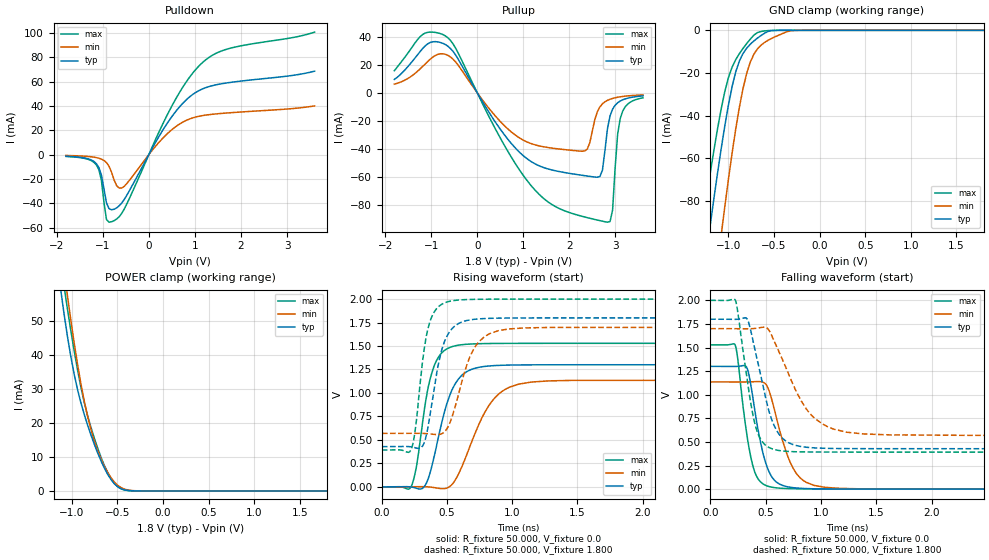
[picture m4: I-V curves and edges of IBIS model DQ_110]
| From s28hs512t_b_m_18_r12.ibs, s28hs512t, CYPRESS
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|   Model DQ_110
[Model] DQ_110
Model_type I/O
Polarity   Non-Inverting
Enable   Active-High
Vinl =  0.630V
Vinh =  1.170V
|Ac timing Thresholds
Vmeas =  0.900V
Cref =  15.000pF
C_comp   5.334pF   5.23pF   5.767pF
[Temperature Range]   25.000   0.125k   -40.000
[Voltage Range]   1.800V   1.700V   2.000V
[Pullup Reference]   1.800V   1.700V   2.000V
[Pulldown Reference]   0.0V   0.0V   0.0V
[POWER Clamp Reference]   1.800V   1.700V   2.000V
[GND Clamp Reference]   0.0V   0.0V   0.0V
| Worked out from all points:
|   slope of the pulldown table from 0 to 0.27 V, typ, clamps not added: 14.9 ohm
|   slope of the pullup table from 0 to 0.27 V, typ, clamps not added: 18.3 ohm
|   GND clamp passes 1 mA (typ) near -0.59 V on its own axis
|   POWER clamp passes 1 mA (typ) near -0.48 V on its own axis
|   rising waveform, R_fixture 50.000, V_fixture 0.0: 20-80 % time 151ps typ, 225ps min, 111ps max; typ from 0 V to 1.3 V
|   rising waveform, R_fixture 50.000, V_fixture 1.800: 20-80 % time 113ps typ, 158ps min, 87.3ps max; typ from 0.428 V to 1.8 V
|   falling waveform, R_fixture 50.000, V_fixture 0.0: 20-80 % time 131ps typ, 181ps min, 109ps max; typ from 1.3 V to 0 V
|   falling waveform, R_fixture 50.000, V_fixture 1.800: 20-80 % time 172ps typ, 292ps min, 127ps max; typ from 1.8 V to 0.428 V
[Pulldown]
|Voltage   I(typ)   I(min)   I(max)
-1.8V     -1.334mA   -724.2uA   -1.502mA
-1.14V    -7.446mA   -2.454mA   -8.441mA
-1.03V    -16.88mA   -3.691mA   -21.21mA
-920mV    -39.73mA   -6.551mA   -53.37mA
-755mV    -44.96mA   -20.8mA    -54.34mA
-645mV    -42.15mA   -27.51mA   -51.1mA
-535mV    -36.94mA   -26.09mA   -44.85mA
510mV     31.81mA    20.83mA    40.71mA
840mV     46.04mA    28.63mA    61.36mA
1.17V     54.13mA    32.13mA    75.91mA
1.775V    59.42mA    34.47mA    87.58mA
3.6V      68.65mA    40.07mA    100.8mA
[Pullup]
|Voltage   I(typ)   I(min)   I(max)
-1.8V     9.461mA    6.095mA    15.71mA
-1.185V   31.57mA    18.73mA    41.62mA
-690mV    34.42mA    27.44mA    40.59mA
575mV     -29.42mA   -23.06mA   -36.75mA
1.29V     -51.46mA   -37.6mA    -70.86mA
2.335V    -59.36mA   -41.64mA   -88.92mA
2.665V    -59.91mA   -10.14mA   -91.51mA
2.83V     -25.5mA    -5.446mA   -92.63mA
2.94V     -11.76mA   -4.09mA    -83.99mA
3.05V     -7.181mA   -3.256mA   -29.58mA
3.105V    -5.964mA   -2.952mA   -18.57mA
3.6V      -2.289mA   -1.585mA   -3.648mA
[GND_clamp]
|Voltage   I(typ)   I(min)   I(max)
-1.8V     -294mA     -373mA     -247.3mA
-1.28V    -116.8mA   -168.5mA   -89.46mA
-1.2V     -91.34mA   -138.7mA   -67.04mA
-1.08V    -55.6mA    -96.11mA   -36.91mA
-1.04V    -44.83mA   -82.66mA   -28.74mA
-1V       -34.98mA   -69.76mA   -22.14mA
-920mV    -19.48mA   -46.23mA   -13.73mA
-800mV    -8.377mA   -20.18mA   -6.205mA
-680mV    -3.579mA   -8.59mA    -1.029mA
-560mV    -408.3uA   -4.544mA   -113.8uA
-280mV    -162.8nA   -73.51uA   -82.13nA
1.8V      272.8pA    325nA      188.3pA
[POWER_clamp]
|Voltage   I(typ)   I(min)   I(max)
-1.8V     236.7mA    239.1mA    251.1mA
-1.123V   59.68mA    73.25mA    67.66mA
-1.086V   52.46mA    65.42mA    60.6mA
-1.049V   45.83mA    57.89mA    53.9mA
-938mV    30.03mA    37.57mA    35.87mA
-864mV    22.62mA    26.6mA     26.18mA
-790mV    16.52mA    18.14mA    18.76mA
-716mV    11.21mA    11.92mA    12.63mA
-642mV    6.708mA    7.258mA    7.47mA
-494mV    1.178mA    1.619mA    1.205mA
-272mV    6.291uA    28.11uA    4.439uA
1.8V      0A         0A         0A
[Ramp]
| variable   typ   min   max
dV/dt_r   0.780/0.151n   0.681/0.226n   0.917/0.110n
dV/dt_f   0.823/0.172n   0.678/0.291n   0.965/0.127n
R_load = 50.000
[Rising Waveform]
R_fixture= 50.000
V_fixture= 0.0
V_fixture_min= 0.0
V_fixture_max= 0.0
|time   V(typ)   V(min)   V(max)
0s        3.146uV    3.895uV    4.875uV
224ps     -849.4uV   1.136mV    1.352mV
265ps     -14.68mV   1.83mV     212.3mV
327ps     6.255mV    1.798mV    833.5mV
418ps     427.3mV    -11.2mV    1.341V
497ps     880.5mV    -13.8mV    1.468V
570ps     1.115V     89.72mV    1.505V
839ps     1.289V     902.2mV    1.527V
1.149ns   1.3V       1.117V     1.528V
6ns       1.301V     1.136V     1.529V
[Rising Waveform]
R_fixture= 50.000
V_fixture= 1.800
V_fixture_min= 1.700
V_fixture_max= 2.000
|time   V(typ)   V(min)   V(max)
0s        428.4mV    569.7mV    392.4mV
221ps     426.8mV    570.6mV    388.3mV
255ps     416.6mV    570.6mV    592.9mV
315ps     440.2mV    569.2mV    1.368V
390ps     939.7mV    560.9mV    1.833V
462ps     1.472V     567.7mV    1.946V
537ps     1.683V     740.2mV    1.981V
717ps     1.786V     1.496V     1.997V
975ps     1.798V     1.682V     1.999V
6ns       1.8V       1.7V       2V
[Falling Waveform]
R_fixture= 50.000
V_fixture= 0.0
V_fixture_min= 0.0
V_fixture_max= 0.0
|time   V(typ)   V(min)   V(max)
0s        1.301V     1.136V     1.529V
224ps     1.3V       1.135V     1.532V
327ps     1.296V     1.135V     615.6mV
413ps     760.7mV    1.139V     151.7mV
481ps     362.1mV    1.131V     52.95mV
550ps     142.4mV    976.3mV    22.56mV
690ps     27.39mV    382.4mV    7.063mV
772ps     13.07mV    177.9mV    4.835mV
1.04ns    2.37mV     19.03mV    2.264mV
6ns       1.812uV    12.99uV    -1.05uV
[Falling Waveform]
R_fixture= 50.000
V_fixture= 1.800
V_fixture_min= 1.700
V_fixture_max= 2.000
|time   V(typ)   V(min)   V(max)
0s        1.8V       1.7V       2V
226ps     1.799V     1.699V     2.005V
334ps     1.802V     1.699V     1.167V
383ps     1.594V     1.7V       805.3mV
437ps     1.311V     1.708V     571.9mV
514ps     905.3mV    1.707V     453.9mV
584ps     658.8mV    1.553V     418.4mV
884ps     442.3mV    826mV      394mV
1.236ns   429.7mV    602.8mV    392.8mV
6ns       428.4mV    569.7mV    392.5mV
